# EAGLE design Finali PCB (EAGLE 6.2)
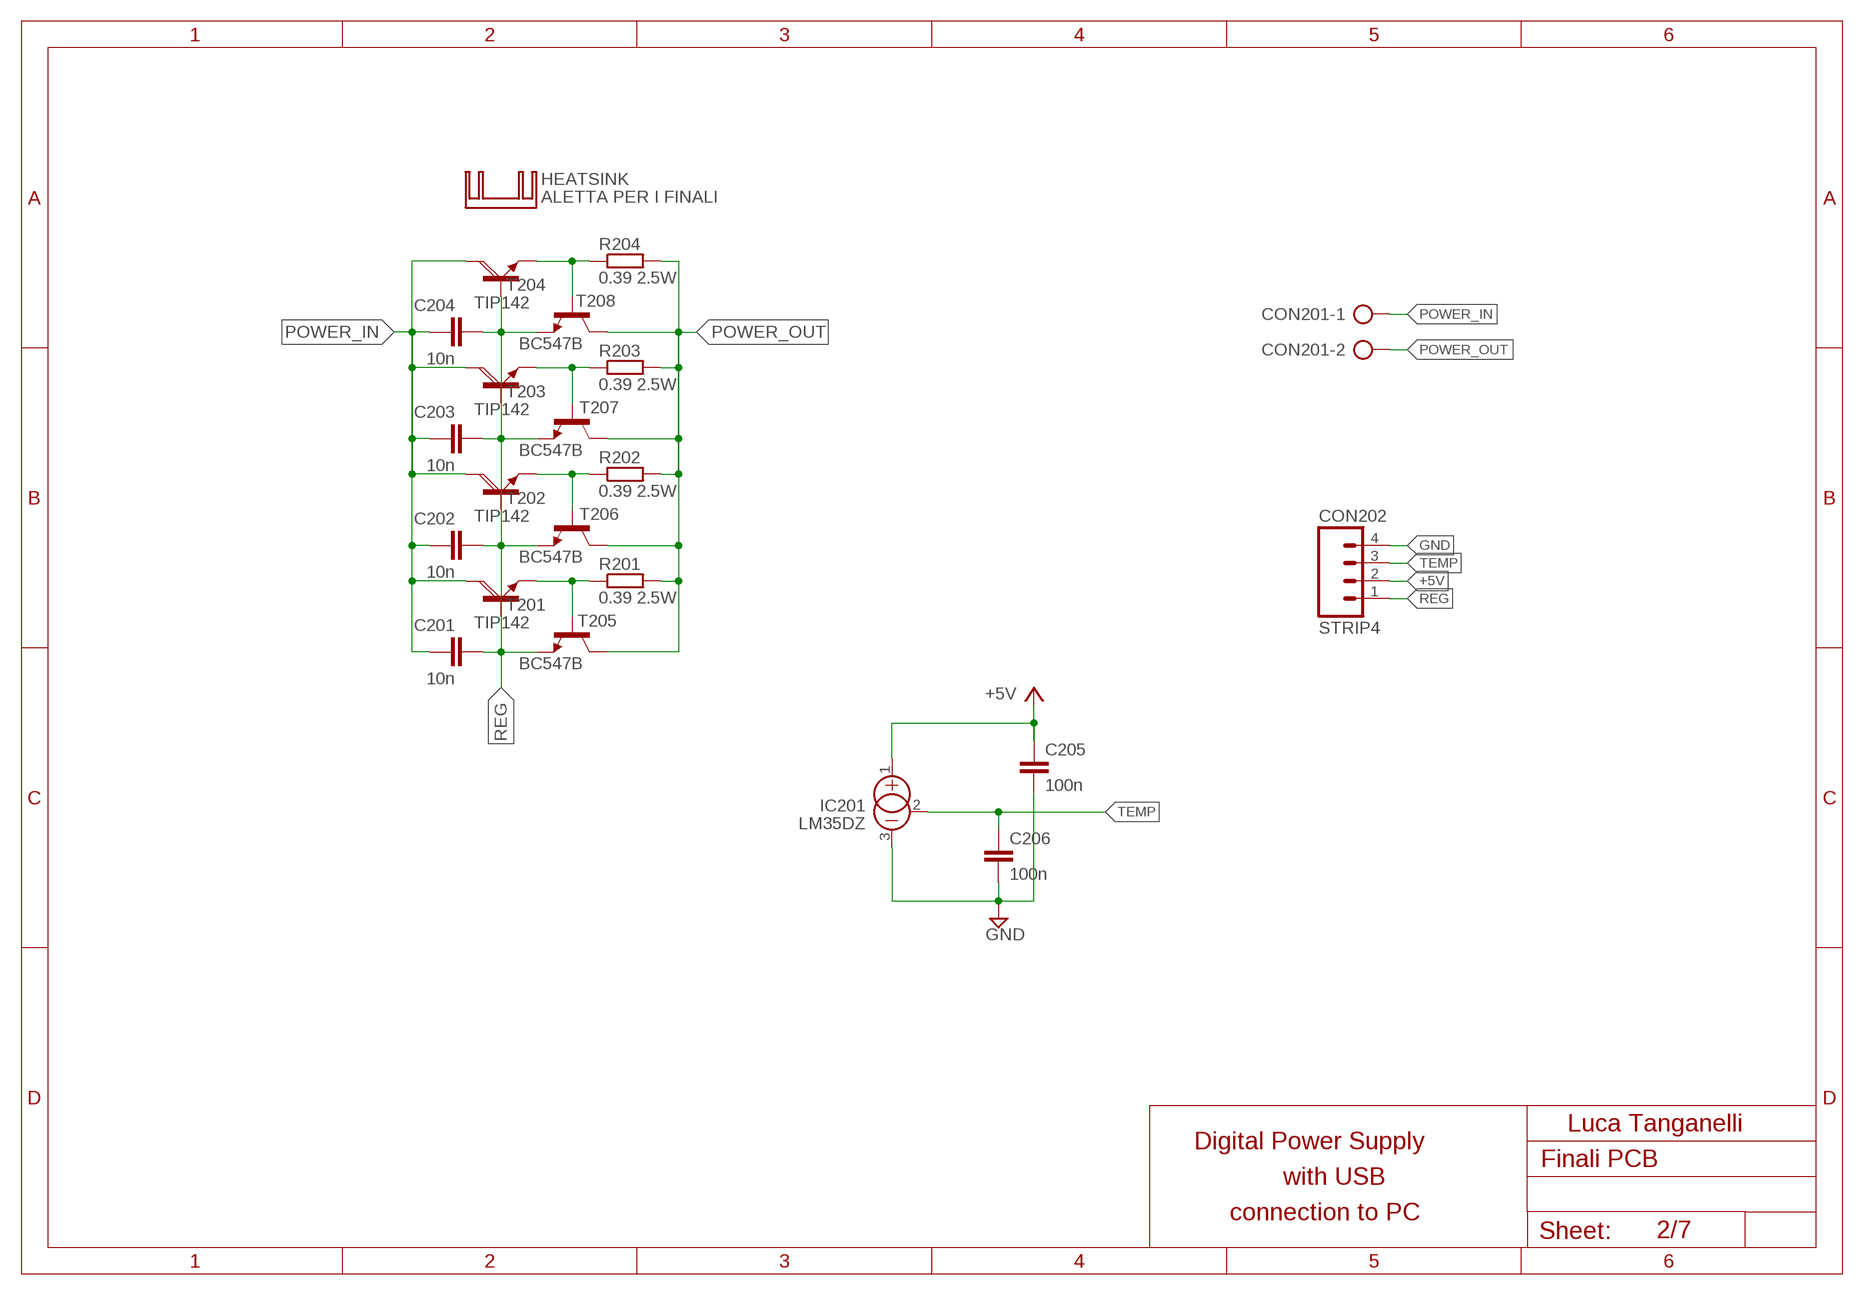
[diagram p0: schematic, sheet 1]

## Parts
C201  10n  C-EU050-024X044  [C050-024X044]
C202  10n  C-EU050-024X044  [C050-024X044]
C203  10n  C-EU050-024X044  [C050-024X044]
C204  10n  C-EU050-024X044  [C050-024X044]
C205  100n  C-EU050-024X044  [C050-024X044]
C206  100n  C-EU050-024X044  [C050-024X044]
CON201  AK500/2  [AK500/2]
CON202  STRIP4  M04  [04P]
HEATSINK  ALETTA PER I FINALI  4TO247  [4TO247]
IC201  LM35DZ  [TO-92]
R201  0.39 2.5W  R-EU_0411/15  [0411/15]
R202  0.39 2.5W  R-EU_0411/15  [0411/15]
R203  0.39 2.5W  R-EU_0411/15  [0411/15]
R204  0.39 2.5W  R-EU_0411/15  [0411/15]
T201  TIP142  [TO247BV]
T202  TIP142  [TO247BV]
T203  TIP142  [TO247BV]
T204  TIP142  [TO247BV]
T205  BC547B  BC547B-NPN-TO92-CBE  [TO92-CBE]
T206  BC547B  BC547B-NPN-TO92-CBE  [TO92-CBE]
T207  BC547B  BC547B-NPN-TO92-CBE  [TO92-CBE]
T208  BC547B  BC547B-NPN-TO92-CBE  [TO92-CBE]

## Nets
+5V: C205.1 CON202.2 IC201.1(+)
GND: C205.2 C206.2 CON202.4 IC201.3(-)
N$38: R204.1 T204.E T208.B
N$39: R203.1 T203.E T207.B
N$40: R202.1 T202.E T206.B
N$41: R201.1 T201.E T205.B
POWER_IN: C201.1 C202.1 C203.1 C204.1 CON201.1 T201.C T202.C T203.C T204.C
POWER_OUT: CON201.2 R201.2 R202.2 R203.2 R204.2 T205.C T206.C T207.C T208.C
REG: C201.2 C202.2 C203.2 C204.2 CON202.1 T201.B T202.B T203.B T204.B T205.E T206.E T207.E T208.E
TEMP: C206.1 CON202.3 IC201.2(CAN)

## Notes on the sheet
- Luca Tanganelli
- Digital Power Supply
- with USB
- connection to PC
- 2/7

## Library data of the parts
C201-C206 = #-rcl:C-EU: CAPACITOR, European symbol
CON201 = #-con-ptr500:AK500/2: CONNECTOR; OC_FARNELL: unknown; OC_NEWARK: unknown
CON202 = #-con-amp-quick:M04: AMP QUICK CONNECTOR; OC_FARNELL: unknown; OC_NEWARK: unknown
HEATSINK = #-heatsink:4TO247
IC201 = #-linear:LM35DZ
R201-R204 = #-rcl:R-EU_: RESISTOR, European symbol
T201-T204 = #-transistor-power:TIP142: NPN DARLINGTON TRANSISTOR
T205-T208 = #-transistor:*-NPN-: NPN Transistror BF959 corrected 2008.03.06

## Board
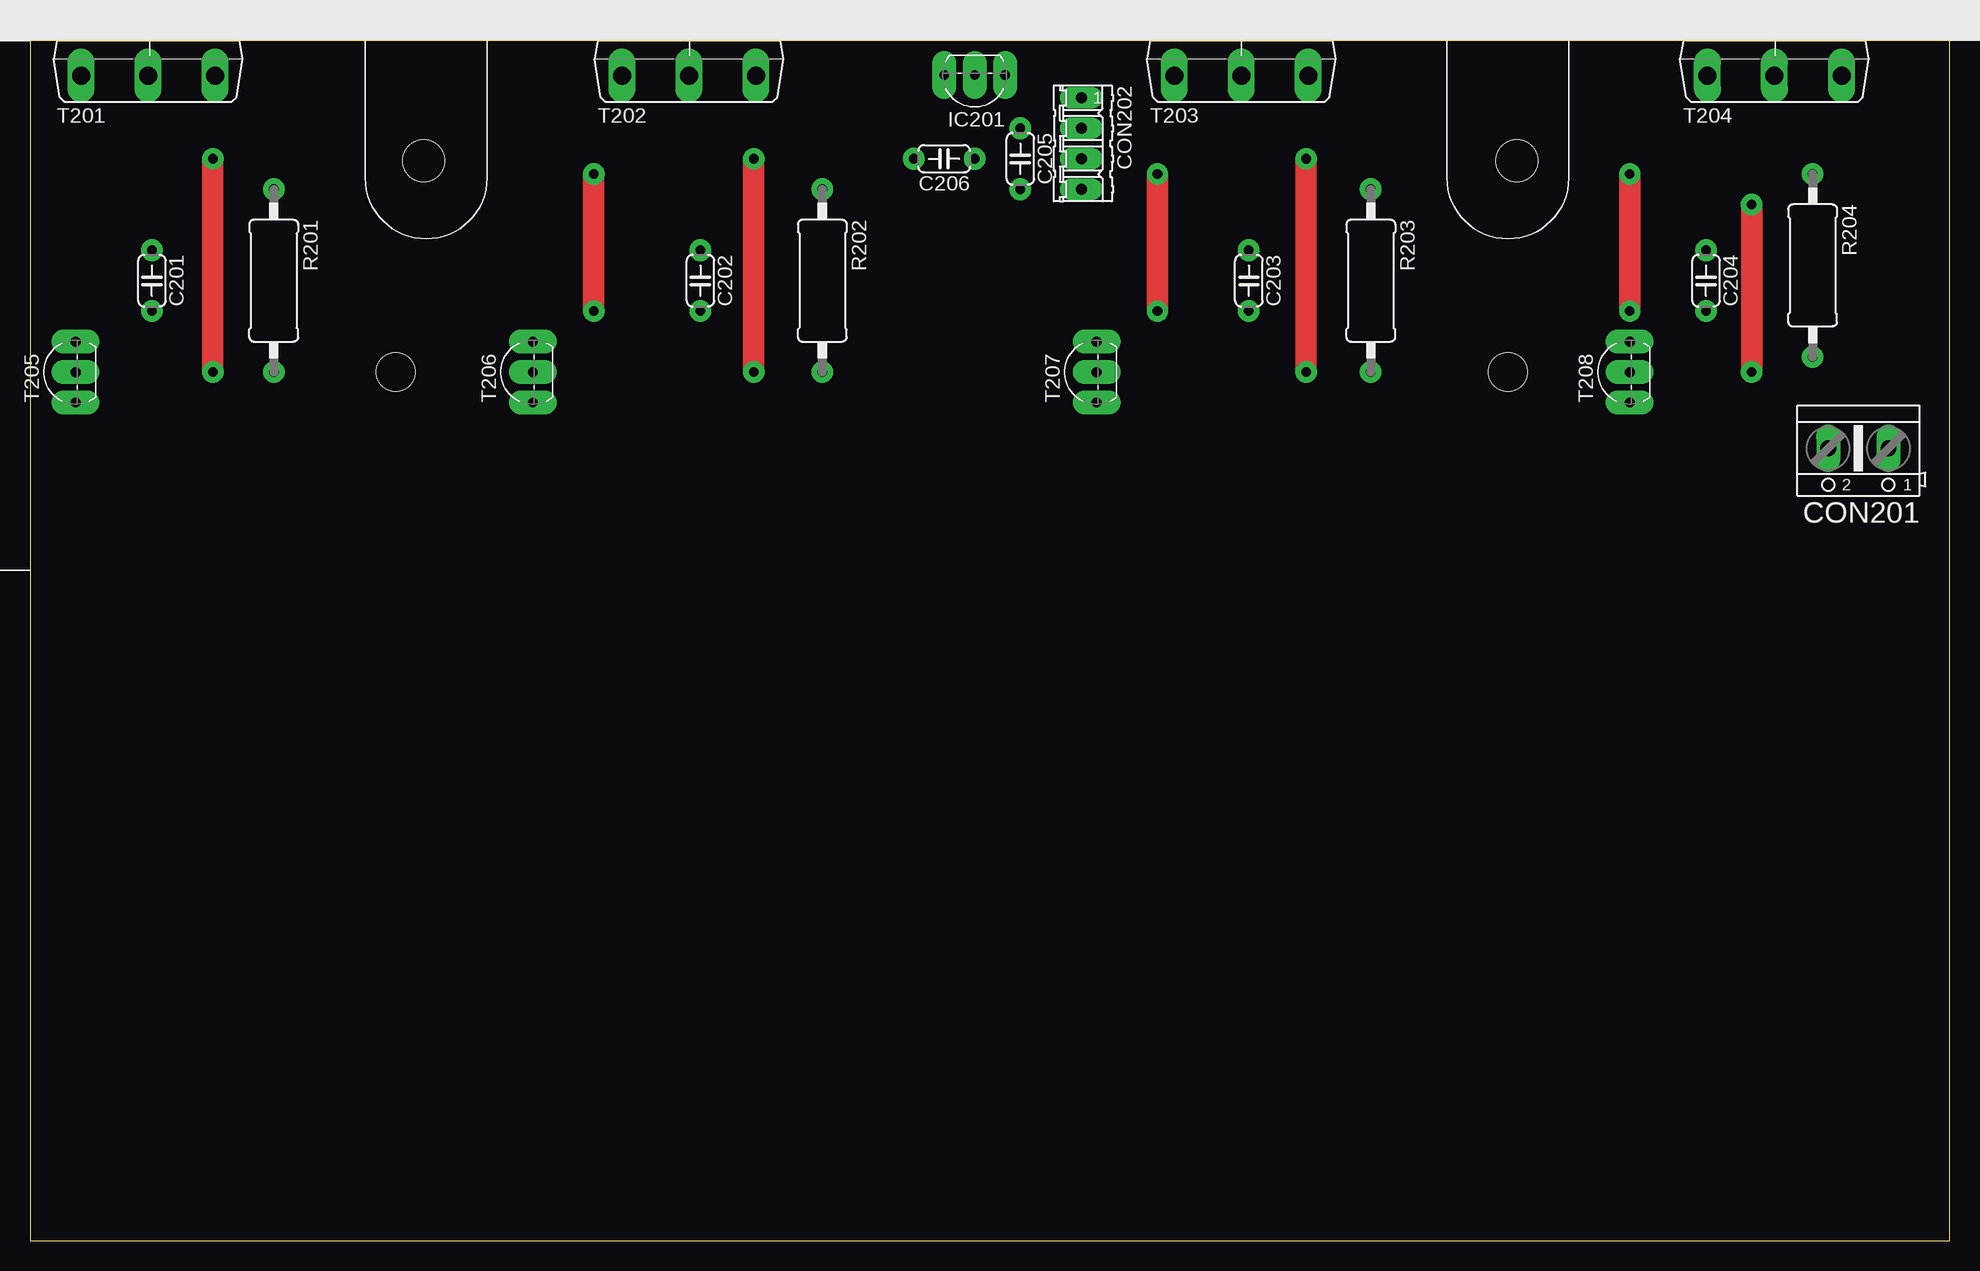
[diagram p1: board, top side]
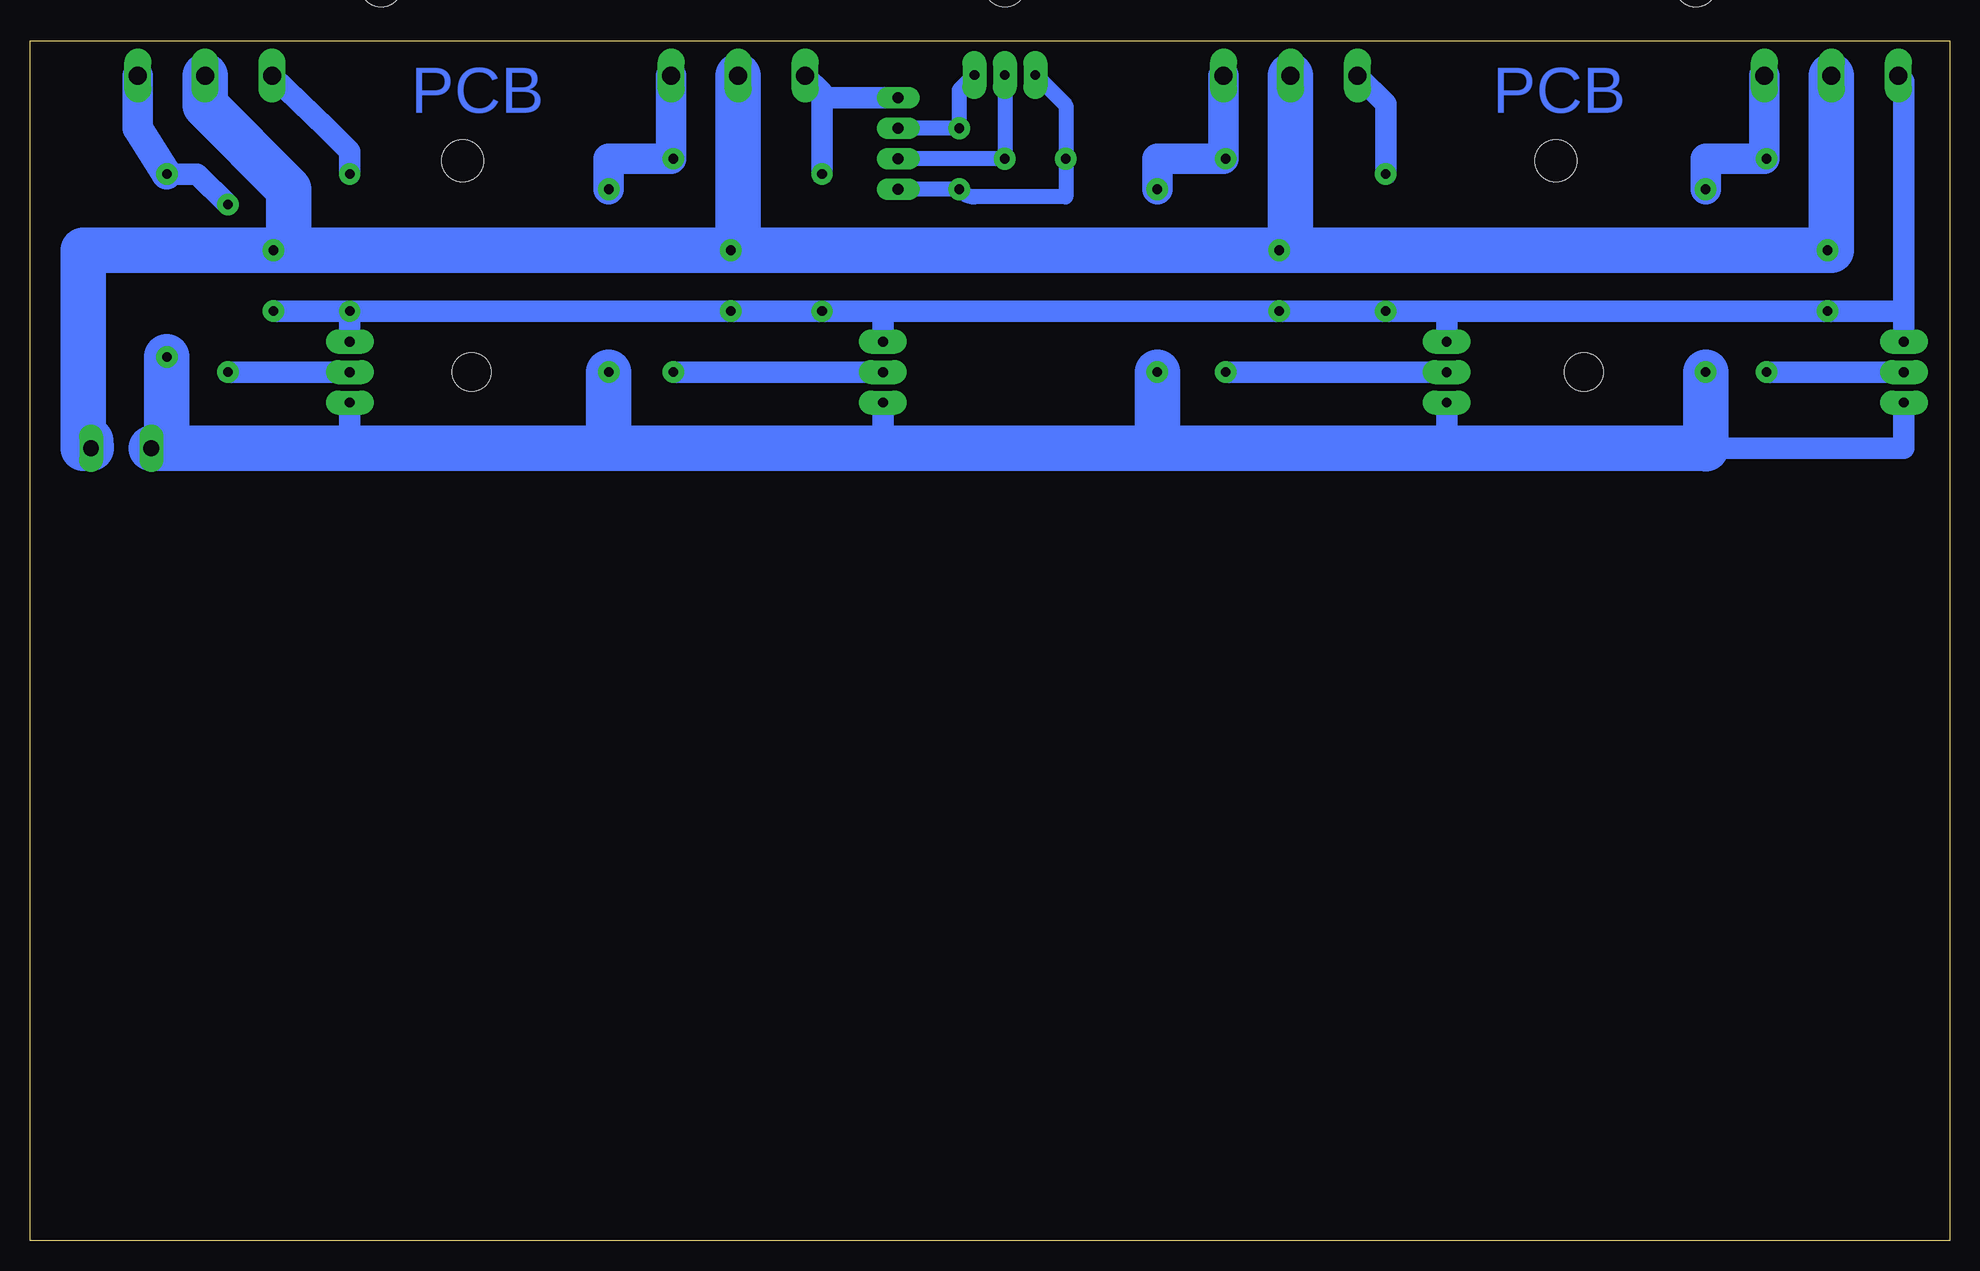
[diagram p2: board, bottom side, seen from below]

Size 160 x 100 mm. Coordinates in mm from the lower left corner, seen from the top.
Outline: 0,0 160,0 160,100 0,100 0,0
Copper layers (1*16): Top 0.035mm / dielectric 1.5mm / Bottom 0.035mm
Design rules: minimum track width 10mil, minimum drill 24mil, track to track 8mil, track to pad 8mil, pad to pad 8mil, via to via 8mil, smd to smd 8mil, copper to edge 40mil, drill to drill 8mil, minimum pad ring 10mil, minimum via ring 8mil, stop-mask expansion 4mil, vias tented up to drill 0mil, thermal gap 10mil
Holes 3.2 mm at 30.48,72.39 123.19,72.39

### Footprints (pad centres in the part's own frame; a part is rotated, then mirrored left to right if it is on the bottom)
C050-024X044 = drill 0.8 pad 1.8: 1 -2.54,0; 2 2.54,0
AK500/2 = drill 1.321 pad 1.7 long: 1 -2.515,0; 2 2.515,0
04P = drill 0.914 pad 1.8 long: 1 -3.81,0; 2 -1.27,0; 3 1.27,0; 4 3.81,0
4TO247 = hole 3.5: 0,4.6; -57.6,4.6; 52,4.6; 91.75,6.5; -91.75,11.5; -45.92,-10; 45.19,-10
TO-92 = drill 0.813 pad 2 long: 1 -2.54,0; 2 0,0; 3 2.54,0
0411/15 = drill 0.8 pad 1.8: 1 -7.62,0; 2 7.62,0
TO247BV = drill 1.499 pad 1.7 long: B -5.588,-2.921; C 0,-2.921; E 5.588,-2.921
TO92-CBE = drill 0.813 pad 2 long: B 0,0; C -2.54,0; E 2.54,0

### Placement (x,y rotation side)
C201  10.16,80.01 270 top
C202  55.88,80.01 270 top
C203  101.6,80.01 270 top
C204  139.7,80.01 270 top
C205  82.55,90.17 270 top
C206  76.2,90.17 180 top
CON201  152.4,66.04 180 top
CON202  87.63,91.44 270 top
HEATSINK  78.74,100.01 0 top
IC201  78.74,97.16 180 top
R201  20.32,80.01 270 top
R202  66.04,80.01 270 top
R203  111.76,80.01 270 top
R204  148.59,81.28 270 top
T201  9.84,100.01 0 top
T202  54.93,100.01 0 top
T203  100.97,100.01 0 top
T204  145.41,100.01 0 top
T205  3.81,72.39 90 top
T206  41.91,72.39 90 top
T207  88.9,72.39 90 top
T208  133.35,72.39 90 top

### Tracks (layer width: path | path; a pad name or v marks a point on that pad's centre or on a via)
+5V
  Bottom 1.27: IC201.1 82.55,95.89 C205.1 CON202.2
GND
  Bottom 1.27: IC201.3 73.66,94.61 C206.2 73.66,87 81.28,87 arc53 C205.2 CON202.4
N$38  (via drill 0.8 pad 1.78)
  Top 1.778: v143.51,72.39 v143.51,86.36
  Bottom 1.778: T208.B v143.51,72.39 | v143.51,86.36 146.05,88.9 R204.1
  Bottom 2.54: T204.E 151,92.71 R204.1
N$39  (via drill 0.8 pad 1.78)
  Top 1.778: v106.36,72.39 v106.36,90.17
  Bottom 1.778: T207.B v106.36,72.39 | v106.36,90.17 106.68,90.17
  Bottom 2.54: T203.E 106.55,90.17 106.68,90.17 111.76,90.17 R203.1
N$40  (via drill 0.8 pad 1.78)
  Top 1.778: v60.33,90.17 v60.33,72.39
  Bottom 1.778: 60.52,90.17 v60.33,90.17 | v60.33,72.39 T206.B
  Bottom 2.54: T202.E 60.52,90.17 66.04,90.17 R202.1
N$41  (via drill 0.8 pad 1.78)
  Top 1.778: v15.24,90.17 v15.24,72.39
  Bottom 1.778: 15.43,90.17 v15.24,90.17 | v15.24,72.39 T205.B
  Bottom 2.54: T201.E 15.43,90.17 20.32,90.17 R201.1
POWER_IN
  Bottom 1.778: 140.34,82.55 146.05,81.92 C204.1 146.05,82.55 | 100.97,82.55 101.6,81.92 C203.1 | 54.93,82.55 55.88,81.6 C202.1 | 9.84,82.55 10.16,82.23 C201.1
  Bottom 3.81: T201.C 9.84,82.55 54.93,82.55 | 54.93,82.55 100.97,82.55 | 100.97,82.55 138.43,82.55 | 138.43,82.55 140.34,82.55 138.43,82.55 | 138.43,82.55 138.43,87.63 145.41,94.61 T204.C | T203.C 100.97,86.36 100.97,82.55 | T202.C 54.93,82.55 | 155.57,66.67 155.57,66.04 155.57,66.67 | 155.57,66.67 155.57,82.55 138.43,82.55 | 138.43,82.55 146.05,82.55 | CON201.1 154.94,66.67 155.57,66.67
POWER_OUT
  Bottom 1.778: T206.C 41.91,66.04 | T205.C 3.81,66.04 13.97,66.04 CON201.2 | T207.C 88.9,66.04 | T208.C 133.35,66.04
  Bottom 3.81: R204.2 148.59,71.12 148.59,66.04 133.35,66.04 111.76,66.04 | 111.76,66.04 R203.2 | R202.2 66.04,66.04 | 66.04,66.04 88.9,66.04 111.76,66.04 | R201.2 20.32,66.04 | 20.32,66.04 41.91,66.04 66.04,66.04 | CON201.2 20.32,66.02 20.32,66.04
REG  (via drill 0.8 pad 1.78)
  Top 1.778: v133.35,88.9 v133.35,77.47 | v93.98,88.9 v93.98,77.47 | v46.99,88.9 v46.99,77.47
  Bottom 1.778: T201.B 3.81,96.65 3.81,77.47 | 3.81,77.47 T205.E 3.81,77.47 | 3.81,77.47 C201.2 41.91,77.47 | 41.91,77.47 T206.E | T206.E 41.91,77.47 | 41.91,77.47 45.72,77.47 | 45.72,77.47 v46.99,77.47 | v46.99,77.47 C202.2 88.9,77.47 | 88.9,77.47 T207.E | T207.E 88.9,77.47 | 88.9,77.47 92.71,77.47 | 92.71,77.47 v93.98,77.47 | v93.98,77.47 C203.2 v133.35,77.47 | v133.35,77.47 T208.E | T208.E v133.35,77.47 | v133.35,77.47 134.62,77.47 | 134.62,77.47 v133.35,77.47 | v133.35,77.47 C204.2 | T204.B 135.25,92.71 133.35,90.81 133.35,89.34 v133.35,88.9 | T203.B 93.98,95.69 93.98,95.25 | 93.98,95.25 v93.98,88.9 | v93.98,77.47 92.71,77.47 | CON202.1 93.98,95.25 | T202.B 46.99,94.74 v46.99,88.9 | v46.99,77.47 45.72,77.47 | T206.E 41.91,77.47 | 41.91,77.47 45.72,77.47 | T207.E 88.9,77.47 | 88.9,77.47 92.71,77.47 | T208.E v133.35,77.47 | v133.35,77.47 134.62,77.47
TEMP
  Bottom 1.27: IC201.2 C206.1 CON202.3

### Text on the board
Bottom: PCB | PCB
